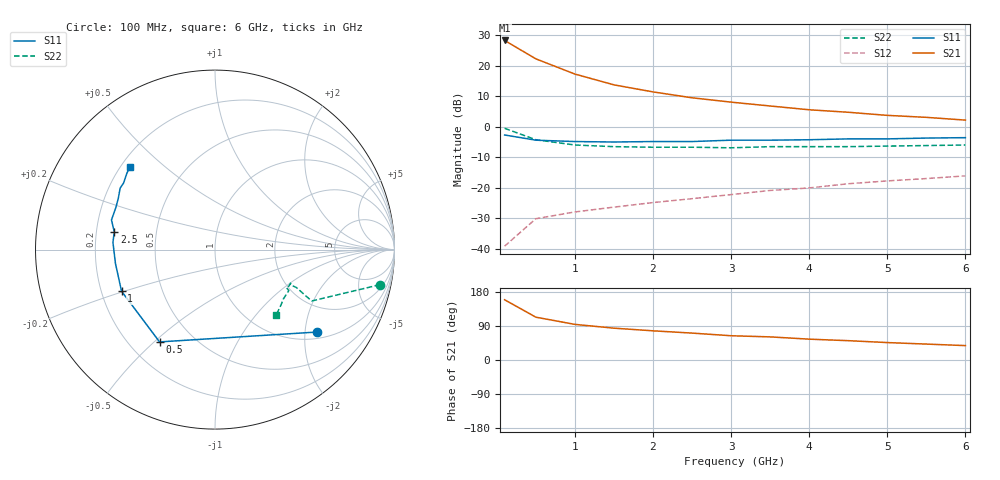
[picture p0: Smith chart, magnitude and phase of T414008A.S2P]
!AT-41400
!S-PARAMETERS at Vce=8V  Ic=10mA.  LAST UPDATED 07-21-92
# ghz s ma r 50
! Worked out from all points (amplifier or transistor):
!   13 points, 100 MHz to 6 GHz, reference 50 ohm
!   highest |S21| = 28.2 dB at 100 MHz (marker M1)
!   |S21| within 3 dB of that: start of sweep to 299.1 MHz
!   unconditionally stable (mu >= 1): 1.463 GHz to 4.564 GHz
!   at 1 GHz: K = 0.78, MSG = 22.6 dB, |S12| = -28.0 dB
!   at 3 GHz: K = 1.14, MAG = 12.9 dB, |S12| = -22.3 dB
!   at 6 GHz: K = 0.88, MSG = 9.1 dB, |S12| = -16.1 dB
!   lowest NFmin = 1.20 dB at 100 MHz
!   S11 on the Smith chart (normalised r, x): 100 MHz: 1.17, -2.31; 500 MHz: 0.32, -0.52; 1 GHz: 0.29, -0.20; 2.5 GHz: 0.28, +0.08; 6 GHz: 0.24, +0.38
0.1  0.73 -39.0  25.84 159.0  0.011 75.0  0.94 -12.0
0.5  0.6 -121.0  12.91 113.0  0.031 48.0  0.61 -28.0
1  0.57 -156.0  7.27 94.0  0.04 51.0  0.5 -25.0
1.5  0.56 -172.0  4.84 84.0  0.048 59.0  0.47 -25.0
2  0.57 176.0  3.71 77.0  0.057 66.0  0.46 -24.0
2.5  0.57 170.0  2.97 71.0  0.066 69.0  0.46 -26.0
3  0.6 164.0  2.52 64.0  0.077 72.0  0.45 -28.0
3.5  0.6 157.0  2.18 61.0  0.09 77.0  0.47 -29.0
4  0.61 152.0  1.89 55.0  0.099 79.0  0.47 -30.0
4.5  0.63 147.0  1.72 51.0  0.116 81.0  0.47 -36.0
5  0.63 144.0  1.53 46.0  0.129 80.0  0.48 -40.0
5.5  0.65 139.0  1.42 42.0  0.141 82.0  0.49 -44.0
6  0.66 136.0  1.28 38.0  0.156 83.0  0.5 -47.0
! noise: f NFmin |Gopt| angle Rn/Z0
0.1  1.2  0.12  3  0.17
0.5  1.2  0.1  15  0.17
1  1.3  0.06  27  0.16
2  1.6  0.24  163  0.16
4  3  0.52  -153  0.18
